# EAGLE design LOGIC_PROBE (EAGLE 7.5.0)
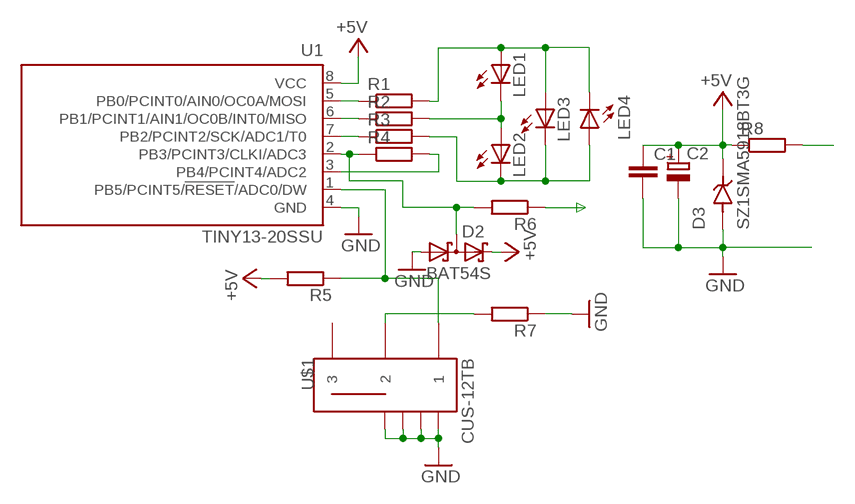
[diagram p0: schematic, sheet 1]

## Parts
C1  C-EUC0603  [C0603]
C2  CPOL-EUSMCC  [SMC_C]
D2  BAT54S  [SOT23]
D3  SZ1SMA5918BT3G  [DIOM5226X220N]
LED1  LEDCHIPLED_0805  [CHIPLED_0805]
LED2  LEDCHIPLED_0805  [CHIPLED_0805]
LED3  LEDCHIPLED_0805  [CHIPLED_0805]
LED4  LEDCHIPLED_0805  [CHIPLED_0805]
R1  R-EU_R0603  [R0603]
R2  R-EU_R0603  [R0603]
R3  R-EU_R0603  [R0603]
R4  R-EU_R0603  [R0603]
R5  R-EU_R0603  [R0603]
R6  R-EU_R0603  [R0603]
R7  R-EU_R0603  [R0603]
R8  R-EU_R2512  [R2512]
U1  TINY13-20SSU  [8S1]
U$1  CUS-12TB  [CUS-12B]

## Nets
+5V: C1.1 C2.+ D2.2(C2) D3.C R5.2 R8.1 U1.8(VCC)
GND: C1.2 C2.- D2.1(A1) D3.A R7.1 U1.4(GND) U$1.P$4(GND) U$1.P$5(GND) U$1.P$6(GND) U$1.P$7(GND)
N$1: D2.3(C1A2) R4.1 R6.2 U1.2(PB3/PCINT3/CLKI/ADC3)
N$2: R4.2 U1.3(PB4/PCINT4/ADC2)
N$3: R1.1 U1.5(PB0/PCINT0/AIN0/OC0A/MOSI)
N$4: R2.1 U1.6(PB1/PCINT1/AIN1/OC0B/INT0/MISO)
N$5: R3.1 U1.7(PB2/PCINT2/SCK/ADC1/T0)
N$7: R5.1 U1.1(PB5/PCINT5/!RESET!/ADC0/DW) U$1.P$1
N$8: R7.2 U$1.P$2
N$11: LED1.A LED3.A LED4.C R1.2
N$12: LED1.C LED2.A R2.2
N$13: LED2.C LED3.C LED4.A R3.2
N$17: R6.1
N$19: R8.2
Unconnected: U$1.P$3

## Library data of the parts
C1 = rcl:C-EU: CAPACITOR, European symbol
C2 = rcl:CPOL-EU: POLARIZED CAPACITOR, European symbol
D2 = diode:BAT54S: Schottky Diodes Pin connection corrected 2011-05-04 Source: Fairchild .. BAT54.pdf
D3 = SZ1SMA5918BT3G:SZ1SMA5918BT3G: Check availability; AVAILABILITY: In Stock; CHECK_PRICES: https://www.snapeda.com/parts/SZ1SMA5918BT3G/Onsemi/view-part/?ref=eda; DESCRIPTION: Zener Diode 5.1 V 1.5 W ±5% Surface Mount SMA; MF: ON Semiconductor; MP: SZ1SMA5918BT3G; PACKAGE: SMA-2 ON Semiconductor; PRICE: None; SNAPEDA_LINK: https://www.snapeda.com/parts/SZ1SMA5918BT3G/Onsemi/view-part/?ref=snap
LED1-LED4 = led:LED: LED
R1-R8 = rcl:R-EU_: RESISTOR, European symbol
U1 = atmel:TINY13: 8-bit AVR Microcontroller with 1K Bytes In-System Programmable Flash Source: http://www.atmel.com/dyn/resources/prod_documents/2535S.pdf; MPN: ATTINY13-20SSU; OC_FARNELL: 1455133; OC_NEWARK: 58M3771
U$1 = CUS-12TB:CUS-12TB: Check availability; AVAILABILITY: In Stock; CHECK_PRICES: https://www.snapeda.com/parts/CUS-12TB/Nidec/view-part/?ref=eda; DESCRIPTION: Slide Switch SPDT Surface Mount, Right Angle; MF: Nidec Copal; MP: CUS-12TB; PACKAGE: None; PRICE: None; SNAPEDA_LINK: https://www.snapeda.com/parts/CUS-12TB/Nidec/view-part/?ref=snap

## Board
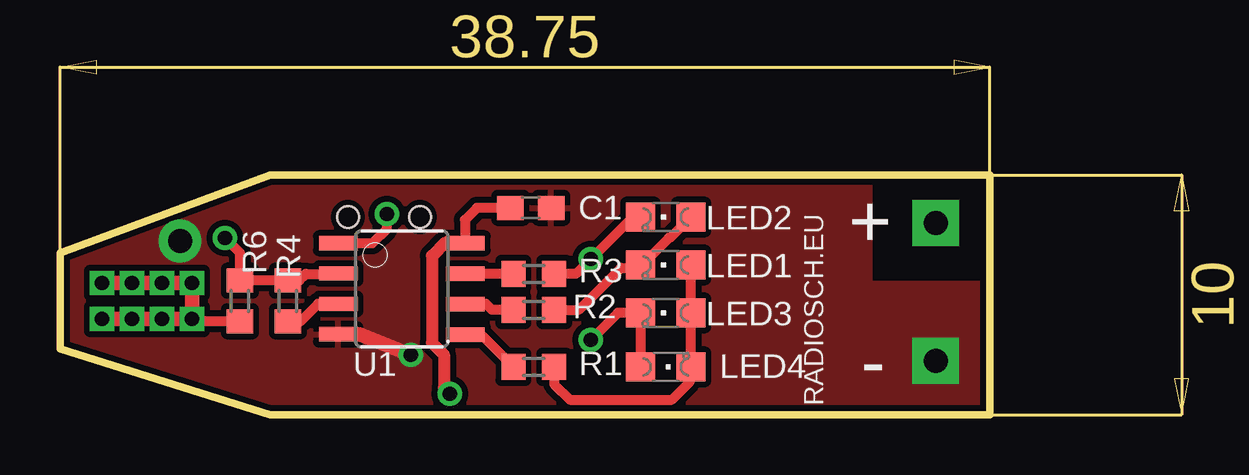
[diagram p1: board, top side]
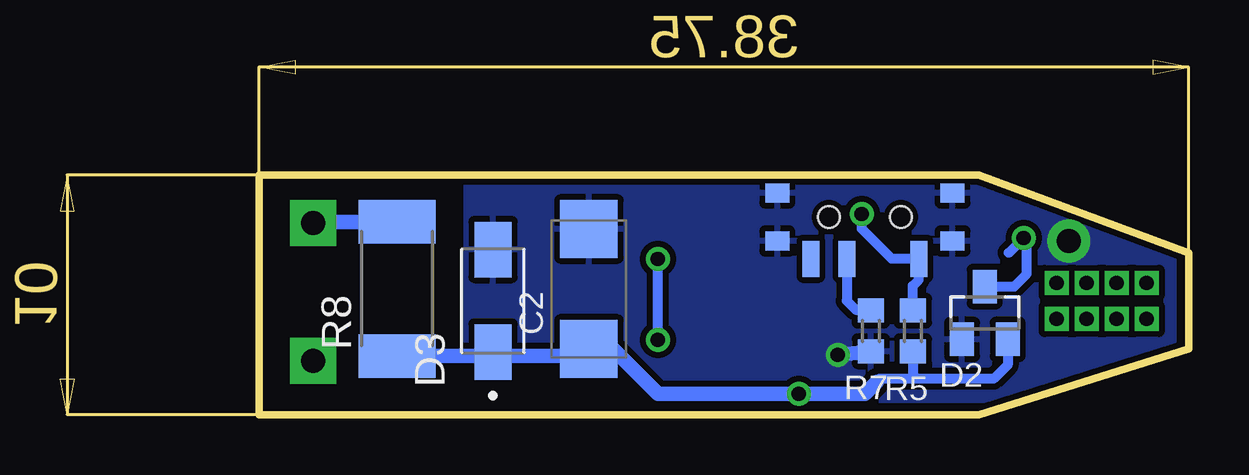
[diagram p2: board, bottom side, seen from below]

Size 47.05 x 14.8 mm. Coordinates in mm from the lower left corner, seen from the top.
Outline: 0,2.75 0,6.75 8.75,10 38.75,10 38.75,0 8.75,0 0,2.75
Copper layers (1*16): Top 0.035mm / dielectric 1.5mm / Bottom 0.035mm
Design rules "default *": minimum track width 10mil, minimum drill 18mil, track to track 8mil, track to pad 8mil, pad to pad 8mil, via to via 8mil, smd to smd 8mil, copper to edge 5mil, drill to drill 8mil, minimum pad ring 10mil, minimum via ring 8mil, stop-mask expansion 2mil, vias tented up to drill 0mil, thermal gap 10mil
tRestrict: area 1.6,4 to 5.6,5.6

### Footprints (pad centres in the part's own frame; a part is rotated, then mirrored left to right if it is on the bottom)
C0603 = smd 1.1 x 1: 1 -0.85,0; 2 0.85,0
SMC_C = smd 2.4 x 2.4: + -2.5,0; - 2.5,0
SOT23 = smd 1 x 1.4: 1 -0.95,-1.1; 2 0.95,-1.1; 3 0,1.1
DIOM5226X220N = smd 2.32 x 1.55: A 2.14,0; C -2.14,0
CHIPLED_0805 = smd 1.2 x 1.2: A 0,-1.05; C 0,1.05
R0603 = smd 1 x 1.1: 1 -0.85,0; 2 0.85,0
R2512 = smd 1.8 x 3.2: 1 -2.8,0; 2 2.8,0
8S1 = smd 0.6 x 1.6: 1 -1.905,-2.654; 2 -0.645,-2.654; 3 0.625,-2.654; 4 1.895,-2.654; 5 1.905,2.654; 6 0.635,2.654; 7 -0.635,2.654; 8 -1.905,2.654
CUS-12B = smd 0.7 x 1.5: P$1 -2.25,1.75; P$2 0.75,1.75; P$3 2.25,1.75 | smd 1 x 0.8: P$4 -3.65,1; P$5 -3.65,-1; P$6 3.65,-1; P$7 3.65,1 | hole 0.9: -1.5,0; 1.5,0

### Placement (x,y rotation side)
C1  19.62,8.62 0 top
C2  25,5.25 90 bottom
D2  8.5,4.25 0 bottom
D3  29,4.75 90 bottom
LED1  25.25,6.25 90 top
LED2  25.25,8.25 90 top
LED3  25.25,4.25 90 top
LED4  25.25,2 270 top
R1  19.75,2 0 top
R2  19.75,4.38 0 top
R3  19.75,5.88 0 top
R4  9.5,4.75 270 top
R5  11.5,3.5 270 bottom
R6  7.5,4.75 90 top
R7  13.25,3.5 90 bottom
R8  33,5.25 90 bottom
U1  14.25,5.25 270 top
U$1  13.5,8.25 180 bottom

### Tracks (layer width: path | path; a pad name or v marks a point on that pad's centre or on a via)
+5V  (via drill 0.6)
  Top 0.406: C1.1 17.38,8.62 16.88,8.12 16.88,7.18 U1.8
  Top 0.5: 16.88,7.18 16.06,7.18 15.5,6.62 15.5,3 16,2.5 16,1.12 v16.25,0.88
  Bottom 0.406: R8.1 29.91,2.45 D3.C | D2.2 7.55,2.08 8.12,1.5 11.38,1.5 | 11.38,1.5 12.88,1.5 13,1.38 | R5.2 11.5,1.62 11.38,1.5
  Bottom 0.61: R8.1 25.3,2.45 C2.+ 24,2.75 22.12,0.88 v16.25,0.88 13.5,0.88 13,1.38
GND  (via drill 0.6, 1 pad 1.78, 1 pad 1.93)
  Top 0.61: U1.4 12.48,3.35 v14.62,2.5
  Bottom 0.61: v14.62,2.5 R7.1
  other vias: 36.5,2.25 5,7.25
  pour Top (isolate 0.254): -2.25,10 33.75,10 33.75,5.5 38.75,5.5 38.75,-0.5 -2.25,-2
  pour Bottom (isolate 0.254): 0.75,9.62 30.12,9.62 30.12,0.62 0.62,0.62 0.62,9.62
N$1  (via drill 0.6)
  Top 0.406: U1.2 11.58,5.88 10.25,5.88 9.97,5.6 R4.1 R6.2 7.5,6.75 v6.88,7.38
  Bottom 0.406: D2.3 7.28,5.35 6.75,5.88 6.75,7.25 v6.88,7.38 7.5,6.75
N$2
  Top 0.406: U1.3 10.75,4.62 10,3.88 9.53,3.88 R4.2
N$3
  Top 0.406: U1.5 17.55,3.35 R1.1
N$4
  Top 0.406: R2.1 18,4.38 17.75,4.62 16.91,4.62 U1.6
N$5
  Top 0.406: U1.7 R3.1
N$7  (via drill 0.6)
  Top 0.406: U1.1 13.03,7.16 13.62,7.75 v13.62,8.38
  Bottom 0.406: R5.1 11.5,5.38 11.25,5.62 U$1.P$1 12.38,6.5 13.62,7.75 v13.62,8.38
N$8
  Bottom 0.406: U$1.P$2 14.25,4.75 13.88,4.38 13.28,4.38 R7.2
N$11
  Top 0.406: R1.2 20.6,1.27 21.25,0.62 25.5,0.62 26.25,1.38 26.25,1.95 LED4.C LED3.A LED1.A
N$12
  Top 0.406: LED2.A 25.43,7.38 25.38,7.38 24.25,6.25 LED1.C 24.07,6.12 23.38,6.12 21.62,4.38 R2.2
N$13  (via drill 0.6)
  Top 0.406: LED4.A LED3.C 23.25,4.25 v22.12,3.12 | LED2.C 23.88,8.25 v22.12,6.5 21.5,5.88 R3.2
  Bottom 0.406: v22.12,3.12 v22.12,6.5
N$17  (via drill 0.6)
  Top 0.406: R6.1 5.6,3.9 v5.5,4
  Top 0.61: v1.75,5.5 v3,5.5 v4.25,5.5 v5.5,5.5 v5.5,4 v4.25,4 v3,4 v1.75,4
N$19  (via drill 1 pad 1.93)
  Bottom 0.61: R8.2 36.45,8.05 v36.5,8

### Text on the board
tPlace: RADIOSCH.EU | + | -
